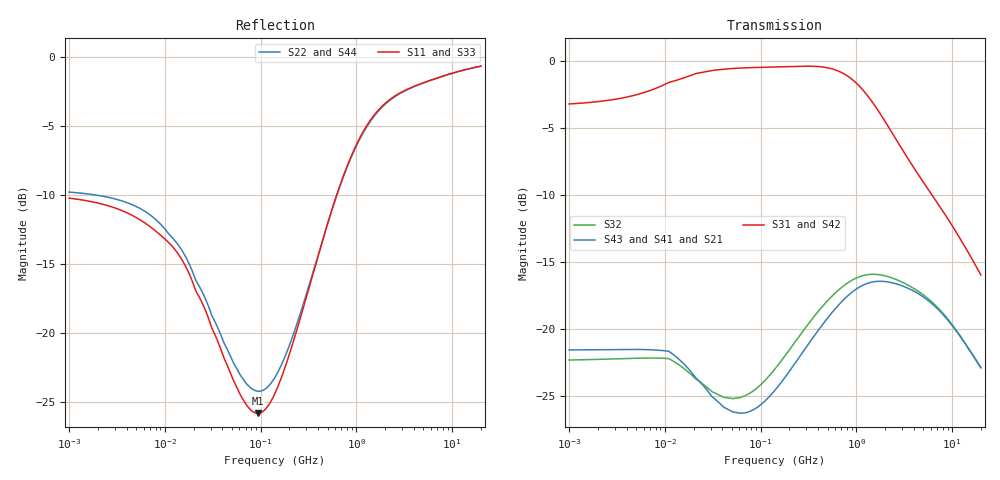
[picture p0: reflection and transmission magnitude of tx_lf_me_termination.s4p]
! Created Wed Jul 29 12:31:03 2015
# hz S db R 50
! 4 Port Network Data from SP1.SP block
! freq  dbS11  angS11  dbS12  angS12  dbS13  angS13  dbS14  angS14
!  dbS21  angS21  dbS22  angS22  dbS23  angS23  dbS24  angS24
!  dbS31  angS31  dbS32  angS32  dbS33  angS33  dbS34  angS34
!  dbS41  angS41  dbS42  angS42  dbS43  angS43  dbS44  angS44
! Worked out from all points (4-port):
!   861 points, 1 MHz to 20 GHz, reference 50 ohm
!   strongest paths, dB at 1 MHz, 11.89 MHz, 141.4 MHz, 1.682 GHz, 20 GHz:
!     S31: -3.2, -1.5, -0.4, -3.6, -16.0
!     S42: -3.4, -1.7, -0.5, -3.7, -16.0
!     S43: -21.6, -21.8, -24.6, -16.4, -22.9
!     S41: -21.6, -21.8, -24.6, -16.4, -22.9
!     S21: -21.6, -21.8, -24.6, -16.4, -22.9
!     S32: -22.3, -22.3, -23.0, -15.9, -22.9
!   lowest |S11| = -25.9 dB at 93.43 MHz (marker M1), VSWR 1.11, Z = 45.2 - j0.63 ohm
!   |S11| at or under -10 dB: start of sweep to 623.4 MHz
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1000000  -10.23 175.2  -22.31 -3.3  -3.18 2.1  -22.31 -3.3
         -21.55 -2.7  -9.79 175.5  -21.55 -2.7  -3.38 2.2
         -3.18 2.1  -22.31 -3.3  -10.23 175.2  -22.31 -3.3
         -21.55 -2.7  -3.38 2.2  -21.55 -2.7  -9.79 175.5
1.189207e7  -13.71 144.4  -22.34 -52.9  -1.51 8.2  -22.34 -52.9
            -21.83 -47.4  -13.08 146.1  -21.83 -47.4  -1.67 8.6
            -1.51 8.2  -22.34 -52.9  -13.71 144.4  -22.34 -52.9
            -21.83 -47.4  -1.67 8.6  -21.83 -47.4  -13.08 146.1
9.342689e7  -25.85 -172.2  -24.35 -137.8  -0.45 -0.4  -24.35 -137.8
            -25.82 -132.1  -24.25 -174.5  -25.82 -132.1  -0.55 -0.4
            -0.45 -0.4  -24.35 -137.8  -25.85 -172.2  -24.35 -137.8
            -25.82 -132.1  -0.55 -0.4  -25.82 -132.1  -24.25 -174.5
4.90506e8  -12.28 -109.3  -17.94 152.3  -0.47 -14.0  -17.94 152.3
           -19.25 149.6  -12.29 -112.5  -19.25 149.6  -0.59 -13.9
           -0.47 -14.0  -17.94 152.3  -12.28 -109.3  -17.94 152.3
           -19.25 149.6  -0.59 -13.9  -19.25 149.6  -12.29 -112.5
1.305408e9  -4.89 -132.4  -15.93 74.9  -2.55 -34.3  -15.93 74.9
            -16.58 71.2  -4.98 -133.3  -16.58 71.2  -2.64 -33.8
            -2.55 -34.3  -15.93 74.9  -4.89 -132.4  -15.93 74.9
            -16.58 71.2  -2.64 -33.8  -16.58 71.2  -4.98 -133.3
3.555088e9  -2.26 -156.3  -16.75 11.9  -7.39 -46.4  -16.75 11.9
            -16.98 10.7  -2.30 -156.4  -16.98 10.7  -7.39 -46.0
            -7.39 -46.4  -16.75 11.9  -2.26 -156.3  -16.75 11.9
            -16.98 10.7  -7.39 -46.0  -16.98 10.7  -2.30 -156.4
2e10  -0.64 -171.5  -22.87 -41.8  -15.96 -59.1  -22.87 -41.8
      -22.89 -41.8  -0.65 -171.5  -22.89 -41.8  -15.95 -59.2
      -15.96 -59.1  -22.87 -41.8  -0.64 -171.5  -22.87 -41.8
      -22.89 -41.8  -15.95 -59.2  -22.89 -41.8  -0.65 -171.5
